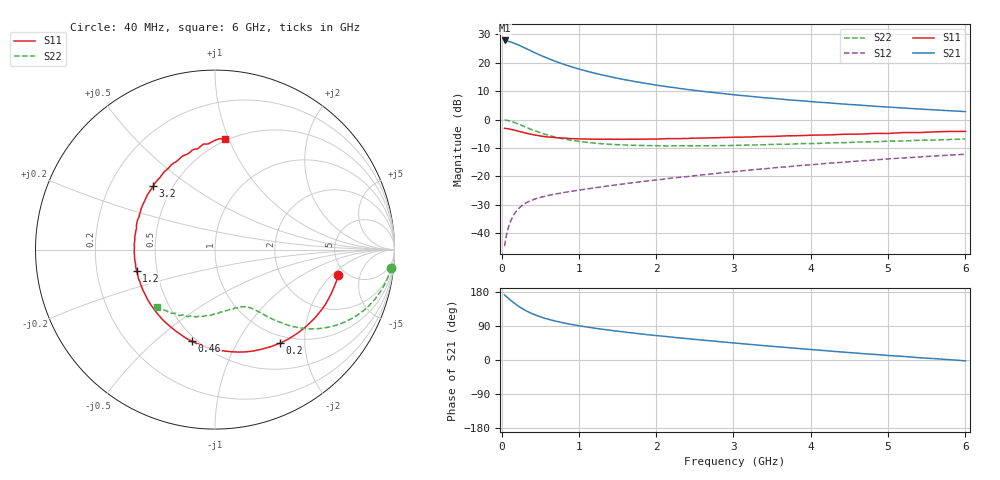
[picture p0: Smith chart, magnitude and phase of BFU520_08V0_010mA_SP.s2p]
! Filename:  P:\Prog\Test\Noise\ATS_data\Testdata_Net\03 Spar\BFU520_APG2013_37_A05_08p0V_010mA_SP_CM01_D.s2p
! Date/Time: Fri 26/Apr/2013 13:00:10
! BFU520_APG2013_37_A05_08p0V_1to20mA_SP_CM01_Bias6_R.s2p
! MDIF S-parameter v. bias file
! BFU520_APG2013_37_A05_08p0V_1to20mA_SP_CM01
! Date/time Tue Apr 23 17:06:44 2013
! VAR V_out= 8.0000
! VAR I_out= 10.0000
! VAR V_in= 0.8266
! VAR I_in= 0.1102
! Device data file deembeded for feedlines and parallel
! Original file: \03 Spar\BFU520_APG2013_37_A05_08p0V_010mA_SP_CM01_R.s2p
! Feed-files: PR047V01_250413_Feed1.s2p, PR047V01_250413_Feed2.s2p
! Parallel-file: PR047V01_250413_Par.s2p
# MHz S MA R 50
!  Freq-MHz  S11-mag  S11-arg  S21-mag  S21-arg  S12-mag  S12-arg  S22-mag  S22-arg
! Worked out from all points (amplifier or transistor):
!   98 points, 40 MHz to 6 GHz, reference 50 ohm
!   highest |S21| = 27.9 dB at 40 MHz (marker M1)
!   |S21| within 3 dB of that: start of sweep to 329.3 MHz
!   unconditionally stable (mu >= 1): 1.837 GHz to 3.852 GHz
!   at 300 MHz: K = 0.30, MSG = 27.4 dB, |S12| = -29.6 dB
!   at 1.6 GHz: K = 0.96, MSG = 18.3 dB, |S12| = -22.6 dB
!   at 6 GHz: K = 0.85, MSG = 7.5 dB, |S12| = -12.2 dB
!   S11 on the Smith chart (normalised r, x): 40 MHz: 4.29, -2.40; 200 MHz: 0.88, -1.54; 460 MHz: 0.47, -0.66; 1.2 GHz: 0.38, -0.11; 3.2 GHz: 0.39, +0.36; 6 GHz: 0.48, +0.97
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40  0.7014 -11.7  24.75 171.8  0.005894 84.0  0.9837 -5.9
50  0.6987 -14.7  24.75 169.3  0.007278 82.6  0.9806 -7.5
60  0.6954 -17.4  24.3 168.1  0.008705 81.5  0.9761 -9.0
120  0.674 -34.6  23.28 157.3  0.01652 74.1  0.9319 -17.4
160  0.6548 -45.2  22.17 150.8  0.02117 69.4  0.8949 -22.3
200  0.6351 -55.1  21.06 144.8  0.02516 65.5  0.852 -26.9
260  0.6045 -69.0  19.41 136.7  0.0302 60.8  0.7895 -32.5
320  0.5757 -81.2  17.78 129.7  0.03423 57.0  0.7299 -37.1
380  0.5522 -91.9  16.21 123.8  0.03745 54.2  0.6755 -40.7
460  0.5264 -104.2  14.42 117.1  0.04109 51.6  0.6153 -44.4
550  0.5027 -116.2  12.75 110.7  0.04415 49.8  0.5569 -47.4
700  0.4807 -131.5  10.57 102.6  0.04889 48.5  0.4913 -50.9
850  0.4671 -143.8  8.98 96.0  0.05312 48.3  0.4452 -53.5
1050  0.4556 -157.1  7.449 88.8  0.0585 48.8  0.4055 -56.3
1200  0.4523 -165.1  6.589 84.1  0.06265 49.4  0.3854 -58.2
1600  0.4494 177.7  5.025 73.5  0.07421 50.9  0.3565 -63.2
2050  0.4568 163.5  3.95 63.5  0.0877 52.1  0.3453 -69.8
3100  0.49 135.9  2.657 43.3  0.1246 51.7  0.3535 -86.6
3200  0.4934 134.4  2.587 41.5  0.129 51.5  0.3561 -87.9
4100  0.5348 115.3  2.024 26.1  0.1642 47.7  0.3805 -103.4
5200  0.5911 96.4  1.597 9.4  0.2111 40.9  0.419 -122.1
6000  0.6193 84.8  1.385 -2.1  0.2454 34.6  0.4555 -135.4
